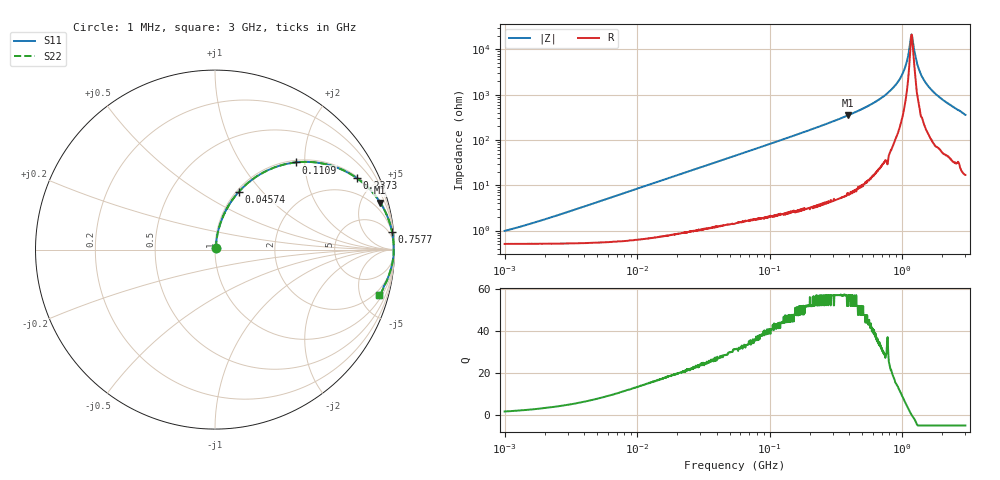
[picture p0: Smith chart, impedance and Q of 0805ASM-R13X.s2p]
!s-Parameter Generated by FASTRON Sdn. Bhd.
!FASTRON P/N : 0805ASM-R13X
!Keysight Technologies: E4991B_MY54100416_A.01.15
!Date: Fri Jun 19 14:50:27 2026
!Version  :Rev00  Fri Jun 19 14:50:27 2026
!Data & Calibration Information:
!Freq  S11  S21  S12  S22
!PortZ  Port1:50+j0  Port2:50+j0
!When reading reference impedance value at option line is always used.
! Remarks : This data is being provided solely for informational purposes.
# Hz S dB R 50
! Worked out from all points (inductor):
!   1601 points, 1 MHz to 3 GHz, reference 50 ohm
!   read as one part in series: L = 134 nH near 1.823 MHz
!   highest Q = 57.3 at 389.5 MHz (marker M1), where L = 142 nH
!   self-resonance near 1.177 GHz
!   S11 on the Smith chart (normalised r, x): 1 MHz: 1.01, +0.02; 45.74 MHz: 1.03, +0.75; 110.9 MHz: 1.04, +1.80; 237.3 MHz: 1.07, +3.96; 757.7 MHz: 2, +20; 3 GHz: 1.34, -7.10
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1000000  -40.20 58.5  -0.04 -0.5  -0.04 -0.5  -40.20 58.5
3804036  -29.80 78.8  -0.05 -1.8  -0.05 -1.8  -29.80 78.8
1.447069e7  -18.50 79.8  -0.12 -6.8  -0.12 -6.8  -18.50 79.8
4.574308e7  -9.20 67.7  -0.67 -20.3  -0.67 -20.3  -9.20 67.7
5.504702e7  -7.85 64.3  -0.90 -23.9  -0.90 -23.9  -7.85 64.3
1.109129e8  -3.58 47.2  -2.69 -41.5  -2.69 -41.5  -3.58 47.2
2.083556e8  -1.33 29.8  -6.06 -59.1  -6.06 -59.1  -1.33 29.8
2.373059e8  -1.05 26.6  -6.98 -62.4  -6.98 -62.4  -1.05 26.6
3.894533e8  -0.39 15.9  -11.20 -73.0  -11.20 -73.0  -0.39 15.9
7.576891e8  -0.07 5.6  -20.20 -82.4  -20.20 -82.4  -0.07 5.6
7.925923e8  -0.06 5.0  -21.30 -82.8  -21.30 -82.8  -0.06 5.0
9.117997e8  -0.05 3.2  -25.00 -82.8  -25.00 -82.8  -0.05 3.2
1.007775e9  -0.04 1.9  -29.30 -81.4  -29.30 -81.4  -0.04 1.9
1.075512e9  -0.04 1.1  -33.80 -77.3  -33.80 -77.3  -0.04 1.1
1.153559e9  -0.04 0.3  -43.70 -46.1  -43.70 -46.1  -0.04 0.3
1.182785e9  -0.04 -0.0  -46.40 7.4  -46.40 7.4  -0.04 -0.0
1.212752e9  -0.04 -0.3  -42.40 48.5  -42.40 48.5  -0.04 -0.3
1.274982e9  -0.04 -0.9  -35.50 74.0  -35.50 74.0  -0.04 -0.9
1.340405e9  -0.04 -1.6  -31.10 79.0  -31.10 79.0  -0.04 -1.6
1.534307e9  -0.06 -3.4  -24.60 81.3  -24.60 81.3  -0.06 -3.4
1.990301e9  -0.14 -7.0  -18.20 79.1  -18.20 79.1  -0.14 -7.0
3e9  -0.44 -15.5  -11.50 71.8  -11.50 71.8  -0.44 -15.5
